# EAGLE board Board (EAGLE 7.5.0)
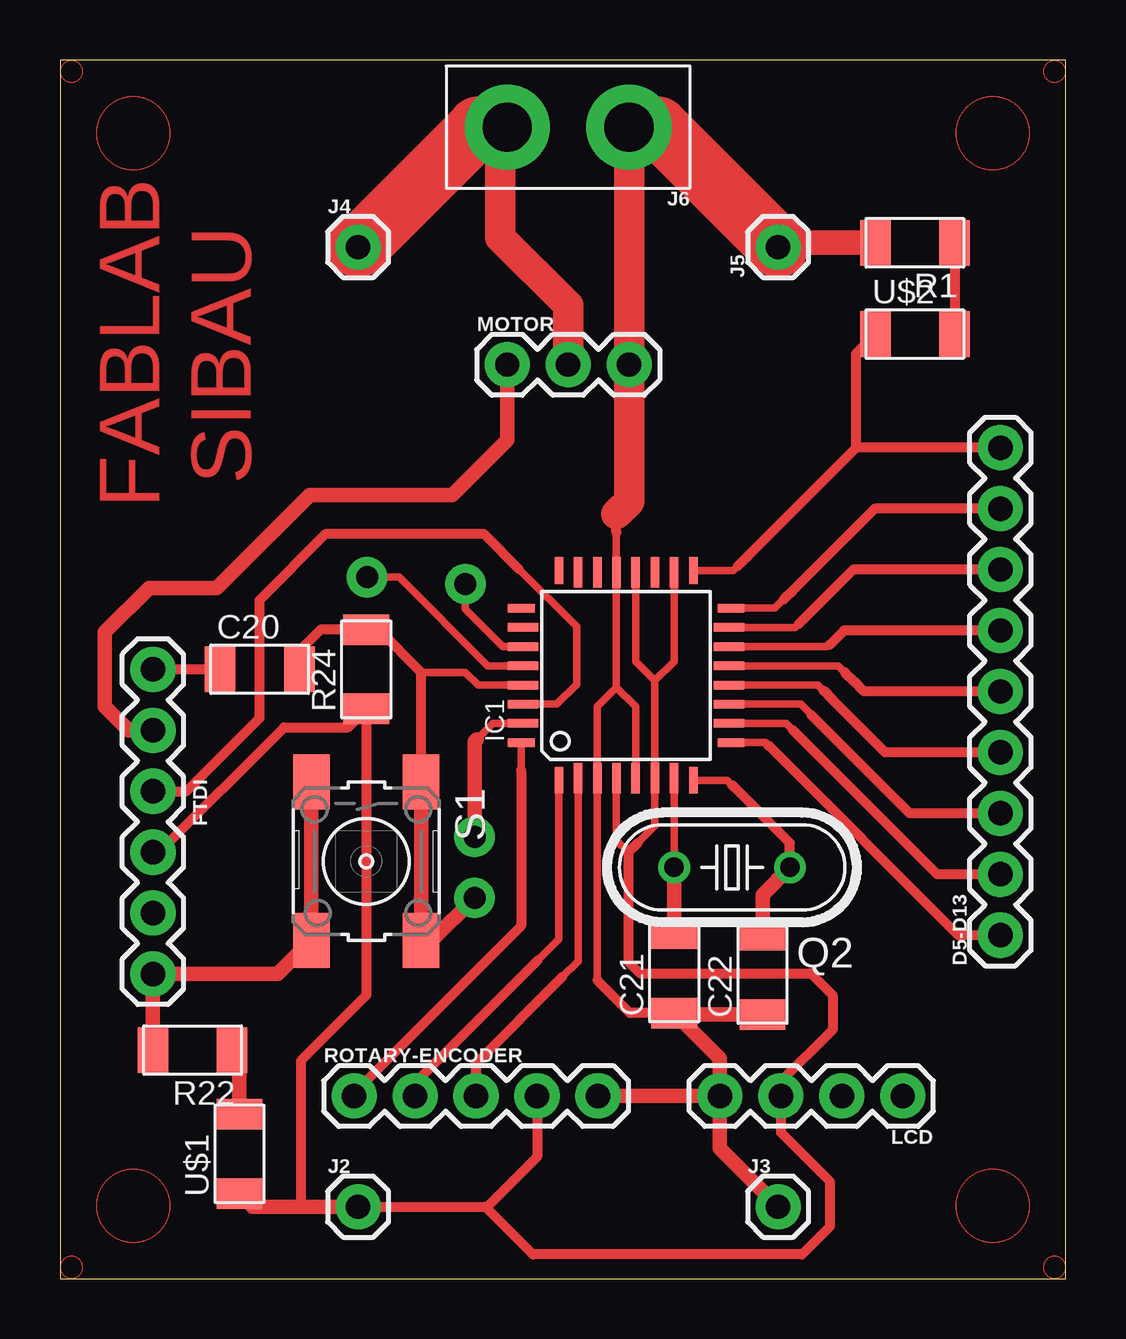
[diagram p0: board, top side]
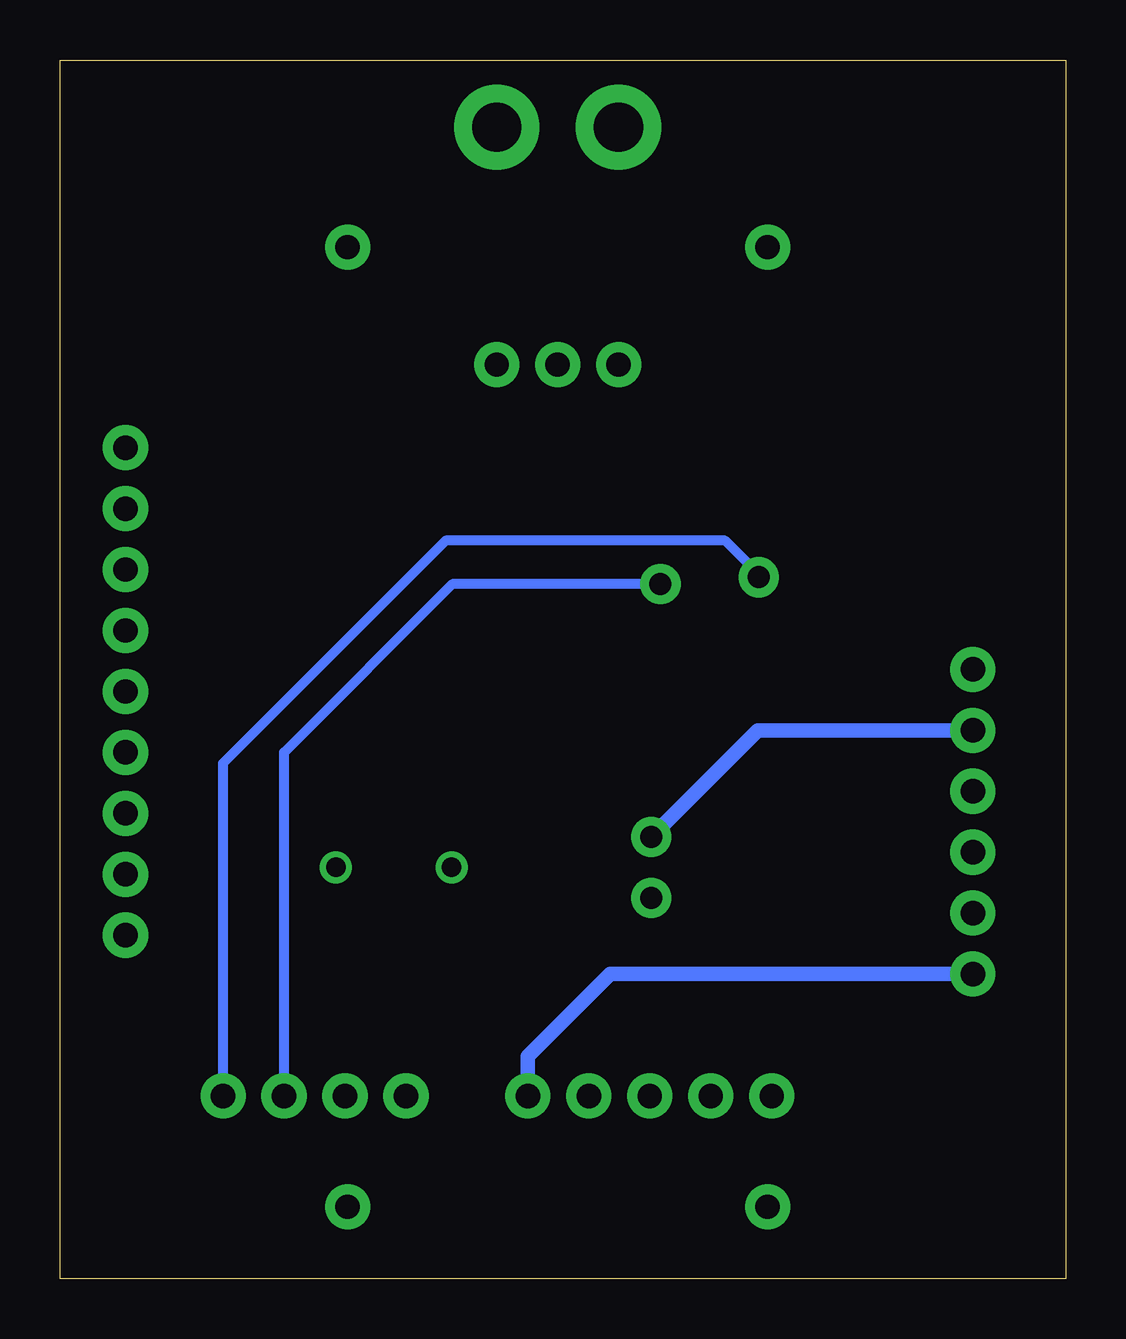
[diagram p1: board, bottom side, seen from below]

Size 41.91 x 50.8 mm. Coordinates in mm from the lower left corner, seen from the top.
Outline: 0,50.8 0,0 41.91,0 41.91,50.8 0,50.8
Copper layers (1*16): Top 0.035mm / dielectric 1.5mm / Bottom 0.035mm
Design rules "default *": minimum track width 10mil, minimum drill 24mil, track to track 12mil, track to pad 12mil, pad to pad 12mil, via to via 12mil, smd to smd 12mil, copper to edge 40mil, drill to drill 8mil, minimum pad ring 10mil, minimum via ring 8mil, stop-mask expansion 4mil, vias tented up to drill 0mil, thermal gap 10mil

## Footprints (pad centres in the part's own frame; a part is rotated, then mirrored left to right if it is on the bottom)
C1206FAB = smd 1.27 x 1.905: 1 -1.651,0; 2 1.651,0
1X09 = drill 1.016 pad 1.88: 1 0,0; 2 2.54,0; 3 5.08,0; 4 7.62,0; 5 10.16,0; 6 12.7,0; 7 15.24,0; 8 17.78,0; 9 20.32,0
FTDI_BASIC = drill 1.016 pad 1.88: CTS 10.16,0; DTR 0,0; GND 12.7,0; RXI 2.54,0; TXO 5.08,0; VCC 7.62,0
TQFP32-08THIN = smd 1.118 x 0.356: 1 -4.369,2.8; 8 -4.369,-2.8; 17 4.369,-2.8; 24 4.369,2.8 | smd 1.27 x 0.356: 2 -4.293,2; 3 -4.293,1.2; 4 -4.293,0.4; 5 -4.293,-0.4; 6 -4.293,-1.2; 7 -4.293,-2; 18 4.293,-2; 19 4.293,-1.2; 20 4.293,-0.4; 21 4.293,0.4; 22 4.293,1.2; 23 4.293,2 | smd 0.356 x 1.118: 9 -2.8,-4.369; 16 2.8,-4.369; 25 2.8,4.369; 32 -2.8,4.369 | smd 0.356 x 1.27: 10 -2,-4.293; 14 1.2,-4.293; 15 2,-4.293; 26 2,4.293; 27 1.2,4.293; 31 -2,4.293 | smd 0.35 x 1.27: 11 -1.2,-4.293; 12 -0.4,-4.293; 13 0.4,-4.293; 28 0.4,4.293; 29 -0.4,4.293; 30 -1.2,4.293
1X01 = drill 1.016 pad 1.88: 1 0,0
1X02_XTRA_BIG = drill 2.057 pad 3.556: 1 -2.54,0; 2 2.54,0
1X04 = drill 1.016 pad 1.88: 1 0,0; 2 2.54,0; 3 5.08,0; 4 7.62,0
1X03 = drill 1.016 pad 1.88: 1 0,0; 2 2.54,0; 3 5.08,0
HC49U-V = drill 0.813: 1 -2.413,0; 2 2.413,0
R1206FAB = smd 1.27 x 1.905: 1 -1.651,0; 2 1.651,0
1X05 = drill 1.016 pad 1.88: 1 0,0; 2 2.54,0; 3 5.08,0; 4 7.62,0; 5 10.16,0
6MM_SWITCH = smd 2.286 x 1.524: 1 -3.302,2.286; 2 3.302,2.286; 3 -3.302,-2.286; 4 3.302,-2.286
LED1206FAB = smd 1.27 x 1.905: 1 -1.651,0; 2 1.651,0

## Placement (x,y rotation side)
C20  0.1uF  [C1206FAB]  8.32,25.4 0 top
C21  22pF  [C1206FAB]  25.59,12.73 90 top
C22  22pF  [C1206FAB]  29.27,12.67 90 top
D5-D13  [1X09]  39.18,14.32 90 top
FTDI  6_PIN_SERIAL_CABLEPTH  [FTDI_BASIC]  3.87,25.4 270 top
IC1  ATMEGA88-THIN  [TQFP32-08THIN]  23.59,25.15 90 top
J2  [1X01]  12.42,3 0 top
J3  [1X01]  29.92,3 0 top
J4  [1X01]  12.42,43 0 top
J5  [1X01]  29.92,43 90 top
J6  [1X02_XTRA_BIG]  21.17,48 180 top
LCD  [1X04]  35.12,7.62 180 top
MOTOR  [1X03]  18.63,38.1 0 top
Q2  [HC49U-V]  28,17.14 180 top
R1  499  [R1206FAB]  35.62,43.18 180 top
R22  499  [R1206FAB]  5.52,9.53 180 top
R24  10k  [R1206FAB]  12.76,25.4 90 top
ROTARY-ENCODER  [1X05]  12.26,7.62 0 top
S1  [6MM_SWITCH]  12.76,17.4 270 top
U$1  pwr led  [LED1206FAB]  7.48,5.21 90 top
U$2  pwr led  [LED1206FAB]  35.62,39.37 0 top

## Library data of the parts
C20-C22 IC1 R1 R22 R24 S1 U$1 U$2 = fab
D5-D13 FTDI J2-J6 ROTARY-ENCODER = SparkFun-Connectors
LCD = SparkFun-Connectors; PROD_ID: CONN-09696
MOTOR = SparkFun-Connectors; PROD_ID: XXX-00000
Q2 = adafruit; OC_FARNELL: 1666969; OC_NEWARK: unknown

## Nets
12VIN: J4.1 J6.2 MOTOR.2
A0: IC1.23
A1: IC1.24
A2: IC1.25
A3: IC1.26
A4: IC1.27 LCD.2
A5: IC1.28 LCD.1
D0: FTDI.TXO IC1.30
D1: FTDI.RXI IC1.31 MOTOR.1
D2: IC1.32 ROTARY-ENCODER.1
D3: IC1.1 ROTARY-ENCODER.2
D4: IC1.2 ROTARY-ENCODER.3
D5: D5-D13.1 IC1.9
D6: D5-D13.2 IC1.10
D7: D5-D13.3 IC1.11
D8: D5-D13.4 IC1.12
D9: D5-D13.5 IC1.13
D10: D5-D13.6 IC1.14
D11: D5-D13.7 IC1.15
D12: D5-D13.8 IC1.16
D13: D5-D13.9 IC1.17 U$2.1
GND: C21.1 C22.1 FTDI.GND IC1.3 IC1.5 IC1.21 J3.1 J5.1 J6.1 LCD.4 MOTOR.3 R1.2 R22.2 ROTARY-ENCODER.5 S1.3 S1.4
N$1: R1.1 U$2.2
N$10: C21.2 IC1.7 Q2.2
N$11: C22.2 IC1.8 Q2.1
N$12: R22.1 U$1.2
N$17: C20.1 FTDI.DTR
RST: C20.2 IC1.29 R24.2 S1.1 S1.2
VCC: FTDI.VCC IC1.4 IC1.6 IC1.18 IC1.20 J2.1 LCD.3 R24.1 ROTARY-ENCODER.4 U$1.1

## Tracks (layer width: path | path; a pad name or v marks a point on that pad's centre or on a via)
12VIN
  Top 1.27: MOTOR.2 21.17,40.58 18.35,43.4 18.35,47.72 J6.2
  Top 2.54: J6.2 17.42,48 J4.1
A4  (via drill 0.91 pad 1.68)
  Top 0.305: IC1.27 18.45,26.35 16.89,27.91 v16.89,28.96
  Bottom 0.406: LCD.2 32.58,21.94 25.56,28.96 v16.89,28.96
A5  (via drill 0.91 pad 1.68)
  Top 0.305: IC1.28 17.82,25.55 14.13,29.24 v12.79,29.24
  Bottom 0.406: LCD.1 35.12,21.5 25.84,30.77 14.19,30.77 12.79,29.37 v12.79,29.24
D0
  Top 0.305: IC1.30 20.71,23.95 21.53,24.77 21.53,27.18 19.11,29.59
  Top 0.406: FTDI.TXO 5.27,20.32 8.32,23.37 8.32,28.29 11.08,31.05 17.65,31.05 19.11,29.59
D1  (via drill 0.91 pad 1.68)
  Top 0.305: IC1.31 18.03,23.15 17.37,22.48
  Top 0.61: v17.27,18.41 17.27,22.38 17.37,22.48 | FTDI.RXI 2.86,22.86 1.87,23.84 1.87,26.96 3.71,28.8 6.54,28.8 10.41,32.67 16.35,32.67 18.63,34.95 MOTOR.1
  Bottom 0.61: FTDI.RXI 12.83,22.86 v17.27,18.41
D2
  Top 0.305: IC1.32 19.22,21.19
  Top 0.406: ROTARY-ENCODER.1 12.26,7.75 19.22,14.71 19.22,21.19
D3
  Top 0.305: IC1.1 20.79,14.15 19.89,13.26 19.53,12.89
  Top 0.406: 19.89,13.26 14.8,8.16 ROTARY-ENCODER.2
D4
  Top 0.305: IC1.2 21.59,13.24 20.92,12.57
  Top 0.406: ROTARY-ENCODER.3 17.34,8.98 20.92,12.57
D5
  Top 0.305: IC1.9 29.41,22.35 29.53,22.23
  Top 0.406: D5-D13.1 37.43,14.32 29.53,22.23
D6
  Top 0.305: IC1.10 30.26,23.15 30.54,22.86
  Top 0.406: D5-D13.2 36.54,16.86 30.54,22.86
D7
  Top 0.305: IC1.11 30.86,23.95 31.69,23.11
  Top 0.406: D5-D13.3 35.4,19.4 31.69,23.11 31.3,23.5
D8
  Top 0.305: IC1.12 31.58,24.75 32.19,24.13
  Top 0.406: D5-D13.4 34.38,21.94 32.19,24.13 31.81,24.51
D9
  Top 0.305: IC1.13 32.43,25.55 33.08,24.89
  Top 0.406: D5-D13.5 33.5,24.48 33.08,24.89 32.7,25.27
D10
  Top 0.305: IC1.14 32,26.35 32.07,26.42
  Top 0.406: D5-D13.6 32.67,27.02 32.07,26.42
D11
  Top 0.305: IC1.15 30.64,27.15 30.99,27.5
  Top 0.406: D5-D13.7 33.05,29.56 30.99,27.5 30.8,27.3
D12
  Top 0.305: IC1.16 29.79,27.95 30.54,28.7
  Top 0.406: D5-D13.8 33.94,32.1 30.54,28.7 30.16,28.32
D13
  Top 0.305: IC1.17 28.05,29.52 28.64,30.1
  Top 0.406: D5-D13.9 33.18,34.64 | 33.18,34.64 28.64,30.1 28.26,29.72 | 33.18,34.64 33.18,38.58 U$2.1
GND
  Top 0.305: 23.19,24.65 IC1.21 23.19,31.11 | 23.19,24.65 22.39,23.85 IC1.3 22.39,12.44 | IC1.5 23.99,23.85 23.19,24.65
  Top 0.406: 23.19,31.11 23.19,31.87 | 22.39,12.44 23.75,11.08 C21.1
  Top 0.61: S1.3 S1.4 9.08,12.7 FTDI.GND R22.2 | LCD.4 ROTARY-ENCODER.5 | LCD.4 27.5,9.18 C21.1 25.65,11.02 C22.1 | LCD.4 27.5,5.43 J3.1
  Top 1.016: R1.2 30.1,43.18 J5.1
  Top 1.27: J6.1 MOTOR.3 23.71,32.4 23.19,31.87
  Top 2.54: J6.1 24.92,48 J5.1
  Bottom 0.61: FTDI.GND 18.99,12.7 22.42,9.27 ROTARY-ENCODER.5
N$1
  Top 0.406: R1.1 U$2.2
N$10
  Top 0.305: IC1.7 Q2.2
  Top 0.61: C21.2 Q2.2
N$11
  Top 0.305: IC1.8 27.8,20.78 28.07,20.51
  Top 0.406: Q2.1 30.42,18.16 28.07,20.51 28,20.57
  Top 0.61: C22.2 29.27,16 Q2.1
N$12
  Top 0.61: U$1.2 7.48,9.22 R22.1
N$17
  Top 0.406: C20.1 FTDI.DTR
RST  (via drill 0.91 pad 1.68)
  Top 0.305: IC1.29 17.42,24.75 16.89,25.27 15.05,25.27
  Top 0.406: C20.2 9.97,26.16 10.86,27.05 R24.2 13.27,27.05 15.05,25.27 S1.1
  Top 0.61: S1.1 S1.2 15.49,14.1 v17.27,15.88
VCC
  Top 0.305: 24.79,24.93 IC1.6 24.79,18.88 24.07,18.16 | 24.79,24.93 23.99,25.73 IC1.20 | IC1.18 25.59,25.73 24.79,24.93 | IC1.4 23.19,18.28 23.69,17.78
  Top 0.406: ROTARY-ENCODER.4 19.88,5.08 17.8,3 17.72,3 | J2.1 17.72,3 | 17.72,3 19.7,1.02 30.92,1.02 32.07,2.16 32.07,4.06 30.04,6.1 LCD.3 30.04,8.22 32.19,10.38 32.19,11.81 31.27,12.73 24.16,12.73 23.69,13.21 23.69,17.78 24.07,18.16 | FTDI.VCC 4.13,17.78 9.34,22.99 12,22.99 R24.1 12.76,11.81 10.03,9.08 10.03,3.1 10.13,3
  Top 0.61: J2.1 10.13,3 8.03,3 U$1.1
(copper drawn outside any net)
  shapes: Top circle x8

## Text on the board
Top: FABLAB / SIBAU

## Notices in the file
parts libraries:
SparkFun-Connectors: Licensing: Creative Commons ShareAlike 4.0 International - https://creativecommons.org/licenses/by-sa/4.0
